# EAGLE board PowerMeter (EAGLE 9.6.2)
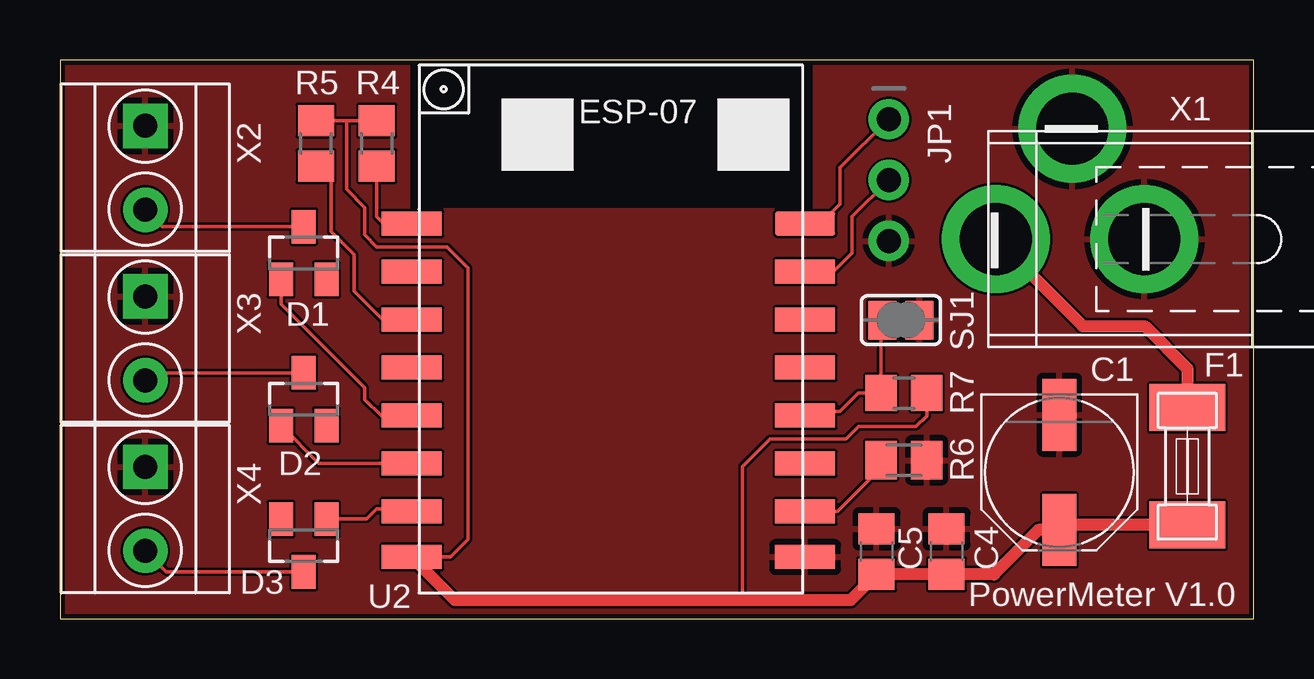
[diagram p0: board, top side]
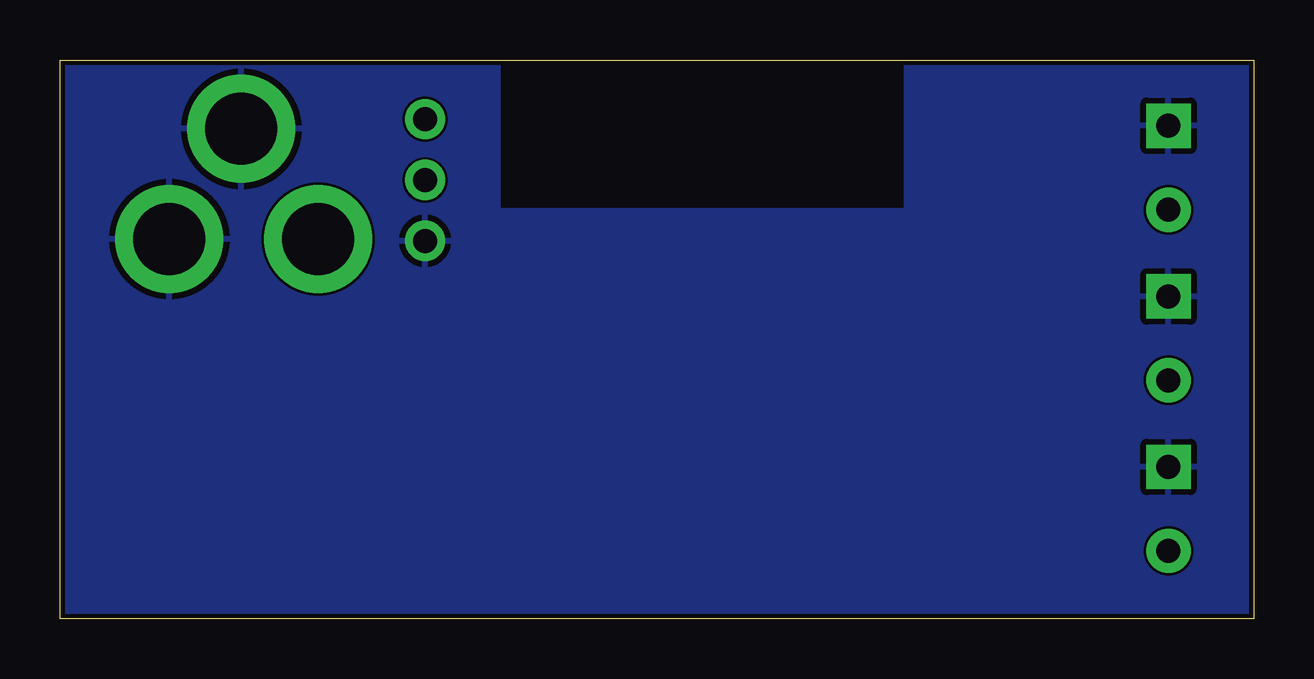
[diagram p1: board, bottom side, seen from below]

Size 49.76 x 23.29 mm. Coordinates in mm from the lower left corner, seen from the top.
Outline: 0,0 49.76,0 49.76,23.29 0,23.29 0,0
Copper layers (1*16): Top 0.035mm / dielectric 1.5mm / Bottom 0.035mm
Design rules "aisler_2_layer": minimum track width 0.1mm, minimum drill 0.2mm, track to track 0.1mm, track to pad 0.1mm, pad to pad 0.1mm, via to via 0.1mm, smd to smd 0.1mm, copper to edge 0.2mm, drill to drill 0.21mm, minimum pad ring 0.25mm, minimum via ring 0.15mm, stop-mask expansion 0mil, vias tented up to drill 0mil, thermal gap 10mil
tRestrict: area 14.6,17.1 to 31.4,23.2
bRestrict: area 14.6,17.1 to 31.4,23.2

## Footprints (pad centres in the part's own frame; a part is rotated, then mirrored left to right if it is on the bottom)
PANASONIC_D = smd 3 x 1.4: + 2.4,0; - -2.4,0
C0805 = smd 1.3 x 1.5: 1 -0.95,0; 2 0.95,0
SOT23 = smd 1 x 1.4: 1 -0.95,-1.1; 2 0.95,-1.1; 3 0,1.1
SMD-6,1X2,6 = smd 1.96 x 3.15: 1 -2.45,0; 2 2.45,0
1X03_ROUND = drill 1 pad 1.676: 1 -2.54,0; 2 0,0; 3 2.54,0
R0805 = smd 1.3 x 1.5: 1 -0.95,0; 2 0.95,0
M0805 = smd 1.3 x 1.6: 1 -0.95,0; 2 0.95,0
SJ = smd 1.168 x 1.6: 1 -0.762,0; 2 0.762,0
ESP07-16PIN = smd 2.5 x 1: ADC -8.2,3.8; CH_PD -8.2,1.8; GND 8.2,-8.105; GPIO0 8.2,-2.2; GPIO2 8.2,-4.2; GPIO4 8.2,1.8; GPIO5 8.2,-0.2; GPIO12 -8.2,-4.2; GPIO13 -8.2,-6.2; GPIO14 -8.2,-2.2; GPIO15 8.2,-6.2; GPIO16 -8.2,-0.2; REST -8.2,5.8; RX 8.2,3.8; TX 8.2,5.8; VCC -8.2,-8.105
HEBW21 = drill 3 pad 4.5: 1 7.5,4.5; 2 10.5,-0.1; 3 13.7,4.5
H2-3.5-7.0X7.0MM = drill 1 pad 1.85 square: 1 -1.75,0 | drill 1 pad 1.85: 2 1.75,0

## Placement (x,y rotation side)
C1  100u/16V  [PANASONIC_D]  41.66,6.1 270 top
C4  100n  [C0805]  36.96,2.79 90 top
C5  10u  [C0805]  34.04,2.79 90 top
D1  BAS70  [SOT23]  10.16,15.24 0 top
D2  BAS70  [SOT23]  10.16,9.14 0 top
D3  BAS70  [SOT23]  10.16,3.05 180 top
F1  T500mA  [SMD-6,1X2,6]  46.99,6.35 270 top
JP1  [1X03_ROUND]  34.54,18.29 270 top
R4  10K  [R0805]  13.21,19.81 270 top
R5  10K  [R0805]  10.67,19.81 270 top
R6  10k  [M0805]  35.18,6.6 0 top
R7  10K  [R0805]  35.18,9.4 0 top
SJ1  [SJ]  35.05,12.45 180 top
U2  ESP07-16PIN  [ESP07-16PIN]  22.86,10.67 0 top
X1  HEBW21  [HEBW21]  52.7,20.32 180 top
X2  GREEN-2P-3.5  [H2-3.5-7.0X7.0MM]  3.56,18.8 270 top
X3  GREEN-2P-3.5  [H2-3.5-7.0X7.0MM]  3.56,11.68 270 top
X4  GREEN-2P-3.5  [H2-3.5-7.0X7.0MM]  3.56,4.57 270 top

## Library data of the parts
C1 C4 C5 = rcl; SPICEPREFIX: C
D1-D3 = diode
F1 = f-lf-omniblok-s
JP1 = microbuilder
R4-R7 = rcl; SPICEPREFIX: R
SJ1 = jumper
U2 = esp8266modules; DIMENSIONS: 22.0 x 16.0 mm; PINS: 16; PITCH: 0.078" / 2 mm
X1 = con-jack
X2-X4 = OPL_Connector

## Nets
+3V3: C1.+ C4.1 C5.1 F1.2 R4.1 R5.1 R7.2 U2.VCC
GND: C1.- C4.2 C5.2 JP1.3 R6.2 SJ1.1 U2.GND X1.1 X1.2 X2.1 X3.1 X4.1
N$1: D1.3 X2.2
N$2: JP1.1 U2.TX
N$3: F1.1 X1.3
N$4: D1.1 U2.GPIO14
N$5: D3.1 U2.GPIO13
N$6: R6.1 U2.GPIO15
N$7: D3.3 X4.2
N$8: D2.1 U2.GPIO12
N$11: JP1.2 U2.RX
N$12: R7.1 SJ1.2 U2.GPIO0
N$14: D2.3 X3.2
N$15: R4.2 U2.REST
N$16: R5.2 U2.CH_PD

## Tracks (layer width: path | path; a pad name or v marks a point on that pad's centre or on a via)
+3V3
  Top 0.152: R4.1 11.94,20.76 | 11.94,20.76 R5.1 | U2.VCC 16.28,2.56 17.02,3.3 17.02,14.61 16.13,15.49 13.21,15.49 12.7,16 12.7,17.14 11.94,17.91 11.94,20.76 | R7.2 36.13,8.44 35.69,8 33.27,8 32.77,7.49 29.59,7.49 28.45,6.35 28.45,0.76
  Top 0.508: F1.2 41.86,3.9 C1.+ 40.78,3.7 38.93,1.84 C4.1 C5.1 32.95,0.76 28.45,0.76 16.46,0.76 U2.VCC
GND
  pour Bottom: 0,23.24 49.78,23.24 49.78,0 0,0
  pour Top: 0,23.24 49.78,23.24 49.78,0 0,0
N$1
  Top 0.152: X2.2 4.26,16.34 D1.3
N$2
  Top 0.152: U2.TX 31.71,16.47 32.51,17.27 32.51,18.8 JP1.1
N$3
  Top 0.5: X1.3 42.63,12.19 45.21,12.19 46.99,10.41 F1.1
N$4
  Top 0.152: D1.1 9.21,13.12 12.7,9.63 12.7,9.14 13.38,8.47 U2.GPIO14
N$5
  Top 0.152: D3.1 12.78,4.15 13.21,4.57 14.56,4.57 U2.GPIO13
N$6
  Top 0.152: U2.GPIO15 32.41,4.47 34.23,6.29 R6.1
N$7
  Top 0.152: D3.3 4.43,1.95 X4.2
N$8
  Top 0.152: U2.GPIO12 10.79,6.47 D2.1
N$11
  Top 0.152: U2.RX 32.25,14.47 33.02,15.24 33.02,16.76 JP1.2
N$12
  Top 0.152: U2.GPIO0 31.23,8.64 32.51,8.64 33.27,9.4 R7.1 34.23,12.38 SJ1.2
N$14
  Top 0.152: D2.3 3.89,10.24 3.58,9.93 X3.2
N$15
  Top 0.152: R4.2 13.21,16.76 13.72,16.26 14.45,16.26 U2.REST
N$16
  Top 0.152: U2.CH_PD 13.44,12.47 12.25,13.65 12.25,15.18 11.3,16.13 11.3,18.23 R5.2

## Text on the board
tNames: PowerMeter V1.0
